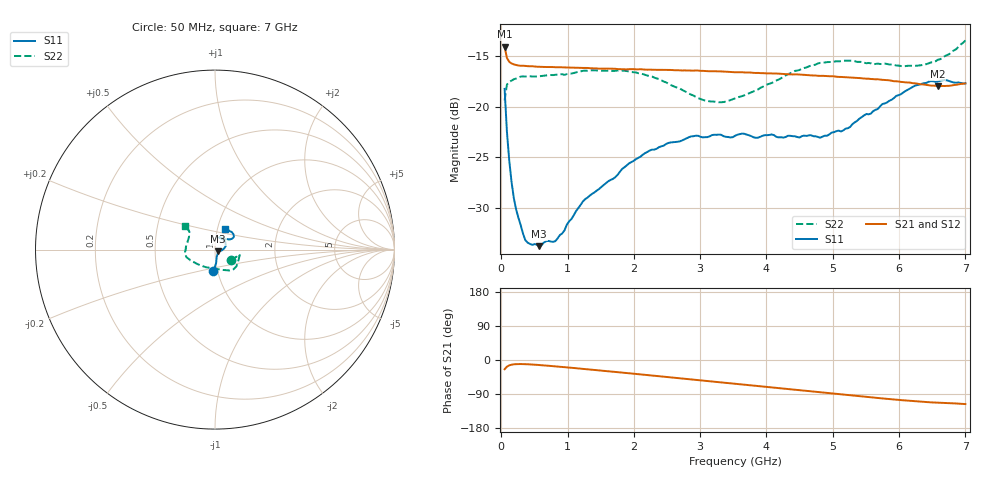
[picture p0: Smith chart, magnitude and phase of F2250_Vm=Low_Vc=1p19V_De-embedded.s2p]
! Integrated Device Technology
! Corporate Headquarters
! 6024 Silver Creek Valley Road
! San Jose, CA 95138  USA
! Phone:  1-408-284-8200
! Toll Free:  1-800-223-1366
! Webpage:  http://www.idt.com/
! Timing and RF Division
! 515 Groton Road, Suite 102
! Westford, MA 01886-6024
! Device:  F2250
! Description: Voltage Variable RF Attenuator
! Frequency:  50.0 -  6000.00 MHz
! Package:  3x3 mm Thin QFN Plastic Package: 16 pin
! Ports:  2 RF, 3 DC
!  Pin  1  = GND
!  Pin  2  = NC
!  Pin  3  = RF1  = Port 1
!  Pin  4  = NC
!  Pin  5  = GND
!  Pin  6  = GND
!  Pin  7  = GND
!  Pin  8  = GND
!  Pin  9  = NC
!  Pin 10  = RF2  = Port 2
!  Pin 11  = NC
!  Pin 12  = GND
!  Pin 13  = GND
!  Pin 14  = VCNTRL
!  Pin 15  = VDD
!  Pin 16  = VMODE
! Vcntrl:  1.190 Volts
! Vmode:  +0.000 Volts
! Vdd:  +3.30  Volts
! Current:  1.192 mA
! Data:  The device was measured on a the F2250 evaluation board which has
!  individual transmission lines to the RF pins.  Data was collected
!  using a calibrated network analyzer.  The evaluation board was
!  de-embedded using a TRL calibration technique.
!  The reference plane is the edge of the package pin.
! Misc:  SN 10
!  Action Tracker AT0258
! Date Measured:  2014-11-26
! Date:  2015-10-15  MJV
! Note:
!  Integrated Device Technology supplies this data as a sample of measured
!  data at the package pin for this product.  Your particular data for this
!  product may vary.
!  Data was taken at 25 degrees C.
!  Integrated Device Technology reserves the right to change this data at anytime.
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# GHz S dB R 50
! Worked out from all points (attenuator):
!   201 points, 50 MHz to 7 GHz, reference 50 ohm
!   highest |S21| = -14.09 dB at 50 MHz (marker M1); lowest = -18.0 dB at 6.583 GHz (marker M2)
!   lowest |S11| = -33.8 dB at 571.2 MHz (marker M3), VSWR 1.04, Z = 51.8 - j0.987 ohm
!   |S11| at or under -10 dB: start of sweep to end of sweep
!   |S22| runs from -19.6 to -13.5 dB; largest |S21 - S12| = 0.00058
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0.05  -18.24 -94.9  -14.09 -24.3  -14.06 -24.3  -19.38 -33.5
0.08475  -22.45 -85.2  -15.18 -17.6  -15.18 -17.6  -17.83 -16.9
0.1195  -25.28 -81.1  -15.57 -14.2  -15.56 -14.2  -17.56 -12.6
0.15425  -27.40 -77.3  -15.73 -12.4  -15.73 -12.4  -17.43 -11.4
0.22375  -30.14 -65.1  -15.89 -10.9  -15.90 -10.9  -17.22 -11.7
0.36275  -33.17 -47.4  -15.97 -11.0  -15.99 -11.0  -17.02 -13.1
0.57125  -33.76 -27.6  -16.05 -13.2  -16.06 -13.2  -17.00 -18.5
0.8145  -33.26 -18.7  -16.10 -16.7  -16.09 -16.7  -16.85 -25.4
1.2315  -29.34 -10.3  -16.17 -23.4  -16.16 -23.4  -16.46 -35.7
1.9265  -25.58 8.6  -16.29 -35.0  -16.29 -35.0  -16.53 -48.5
2.37825  -23.99 19.9  -16.35 -42.7  -16.34 -42.7  -17.27 -58.1
2.86475  -22.93 35.6  -16.44 -51.1  -16.43 -51.1  -18.81 -75.9
3.07325  -23.00 42.6  -16.48 -54.8  -16.48 -54.8  -19.39 -87.3
3.3165  -22.77 51.6  -16.52 -59.1  -16.50 -59.1  -19.56 -103.0
3.525  -22.87 57.0  -16.60 -62.7  -16.59 -62.7  -19.17 -116.3
4.7065  -22.91 65.1  -16.92 -83.4  -16.90 -83.5  -15.91 -163.1
4.81075  -23.06 61.5  -16.96 -85.2  -16.95 -85.3  -15.67 -164.9
5.15825  -22.34 49.3  -17.08 -91.4  -17.08 -91.4  -15.46 -172.3
5.85325  -19.41 33.2  -17.40 -103.1  -17.40 -103.2  -15.84 172.2
6.2355  -17.94 34.1  -17.69 -108.9  -17.69 -109.0  -15.97 159.5
6.583  -17.51 42.1  -17.97 -112.6  -17.95 -112.6  -15.37 147.5
7  -17.69 63.5  -17.70 -116.3  -17.70 -116.4  -13.46 142.6
